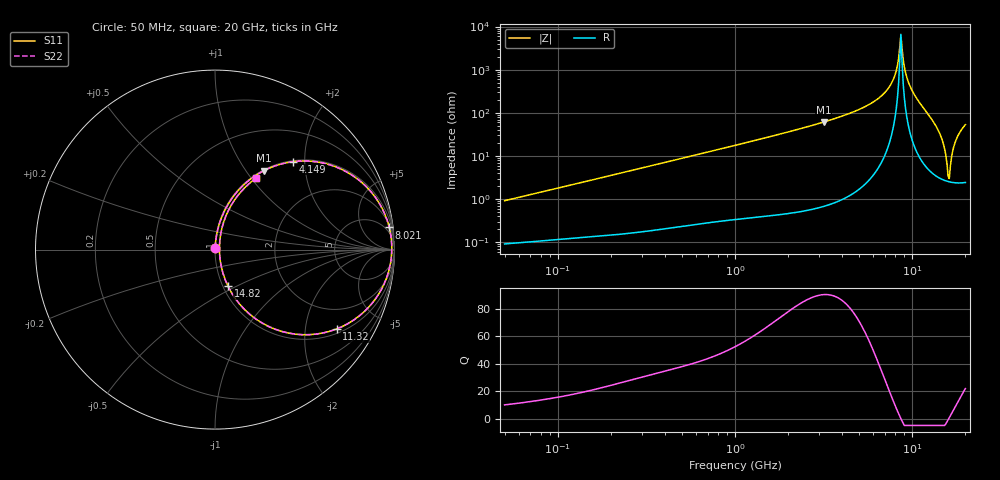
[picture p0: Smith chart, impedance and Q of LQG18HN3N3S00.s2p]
!Murata Part Number: LQG18HN3N3S00
!These Parameters are Measured in Series Mode Connection
!  o--[Z]--o
!Port1  Port2
!  o-------o
!Freq. Start=50[MHz] Stop=20[GHz], 401[Steps]
# Hz S RI R 50
!Freq.(Hz) S11(Real) S11(Imag) S21(Real) S21(Imag) S12(Real) S12(Imag) S22(Real) S22(Imag)
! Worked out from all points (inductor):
!   401 points, 50 MHz to 20 GHz, reference 50 ohm
!   read as one part in series: L = 2.89 nH near 51.52 MHz
!   highest Q = 90.3 at 3.169 GHz (marker M1), where L = 3.07 nH
!   self-resonance near 8.516 GHz
!   S11 on the Smith chart (normalised r, x): 50 MHz: 1.00, +0.02; 4.149 GHz: 1.02, +1.75; 8.021 GHz: 3, +15; 11.32 GHz: 1.15, -2.95; 14.82 GHz: 1.06, -0.45; 20 GHz: 1.05, +1.06
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5e7  0.000996 0.00911  0.999 -0.00911  0.999 -0.00911  0.000996 0.00911
1.364002e8  0.00187 0.0243  0.9981 -0.0243  0.9981 -0.0243  0.00187 0.0243
3.721004e8  0.00622 0.0651  0.9938 -0.0651  0.9938 -0.0651  0.00622 0.0651
1e9  0.033 0.1693  0.967 -0.1693  0.967 -0.1693  0.033 0.1693
2.728004e9  0.2096 0.4014  0.7904 -0.4014  0.7904 -0.4014  0.2096 0.4014
3.168813e9  0.2744 0.4407  0.7256 -0.4407  0.7256 -0.4407  0.2744 0.4407
4.149438e9  0.4358 0.49  0.5642 -0.49  0.5642 -0.49  0.4358 0.49
6.034176e9  0.7557 0.4198  0.2443 -0.4198  0.2443 -0.4198  0.7557 0.4198
7.442007e9  0.9314 0.229  0.0686 -0.229  0.0686 -0.229  0.9314 0.229
8.020766e9  0.9709 0.1237  0.0291 -0.1237  0.0291 -0.1237  0.9709 0.1237
8.389408e9  0.983 0.0514  0.017 -0.0514  0.017 -0.0514  0.983 0.0514
8.644534e9  0.985 -9.95e-05  0.015 9.95e-05  0.015 9.95e-05  0.985 -9.95e-05
8.774992e9  0.9838 -0.0267  0.0162 0.0267  0.0162 0.0267  0.9838 -0.0267
9.178299e9  0.9708 -0.1089  0.0292 0.1089  0.0292 0.1089  0.9708 -0.1089
9.600142e9  0.9417 -0.1925  0.0583 0.1925  0.0583 0.1925  0.9417 -0.1925
1.131968e10  0.677 -0.4423  0.323 0.4423  0.323 0.4423  0.677 -0.4423
1.334722e10  0.2604 -0.4079  0.7396 0.4079  0.7396 0.4079  0.2604 -0.4079
1.482269e10  0.0729 -0.2047  0.9271 0.2047  0.9271 0.2047  0.0729 -0.2047
1.573793e10  0.0288 -0.0583  0.9712 0.0583  0.9712 0.0583  0.0288 -0.0583
1.621653e10  0.0248 0.0154  0.9752 -0.0154  0.9752 -0.0154  0.0248 0.0154
1.774144e10  0.0735 0.2159  0.9265 -0.2159  0.9265 -0.2159  0.0735 0.2159
2e10  0.2308 0.3991  0.7692 -0.3991  0.7692 -0.3991  0.2308 0.3991
